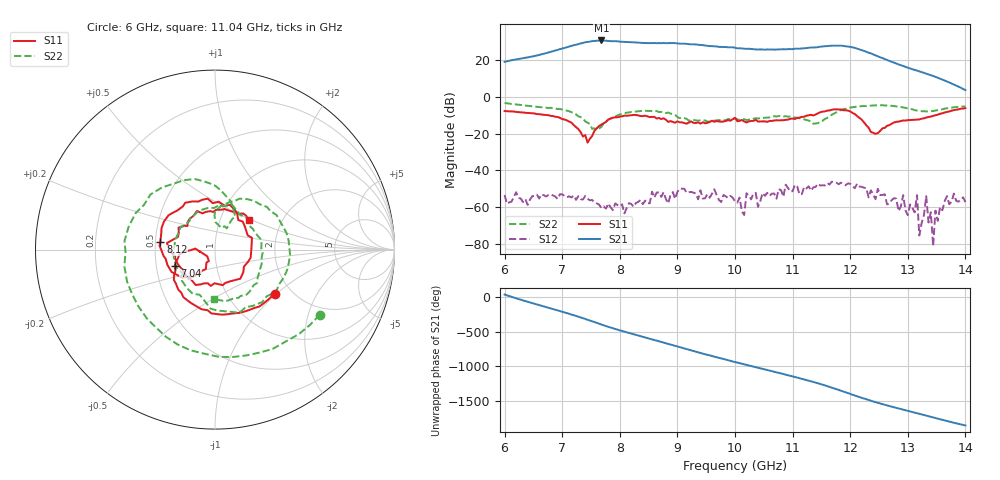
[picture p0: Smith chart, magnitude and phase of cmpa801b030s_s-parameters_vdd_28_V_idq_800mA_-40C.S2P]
!Keysight Technologies,E5071C,MY46110325,B.14.03
!Date: Tue Aug 11 10:33:59 2020
!Data & Calibration Information:
!Freq	S11:SOLT2(ON)	S21:SOLT2(ON)	S12:SOLT2(ON)	S22:SOLT2(ON)
!PortZ  Port1:50+j0  Port2:50+j0
!Above PortZ is port z conversion or system Z0 setting when saving the data.
!When reading, reference impedance value at option line is always used.
# Hz S dB R 50
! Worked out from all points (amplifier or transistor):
!   201 points, 6 GHz to 14 GHz, reference 50 ohm
!   highest |S21| = 30.9 dB at 7.68 GHz (marker M1)
!   |S21| within 3 dB of that: 7.159 GHz to 9.532 GHz (2.373 GHz wide, 28.4 % of centre)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
!   unconditionally stable (mu >= 1): start of sweep to end of sweep
!   at 7.32 GHz: K = 9.67, MAG = 29.7 dB, |S12| = -55.8 dB
!   at 10 GHz: K = 13.75, MAG = 27.5 dB, |S12| = -57.0 dB
!   at 14 GHz: K = 124.67, MAG = 6.6 dB, |S12| = -57.4 dB
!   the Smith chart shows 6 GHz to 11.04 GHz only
!   S11 on the Smith chart (normalised r, x): 6 GHz: 1.64, -0.98; 7.04 GHz: 0.62, -0.12; 8.12 GHz: 0.53, +0.05; 11.04 GHz: 1.36, +0.49
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6e9  -7.63 -36.4  19.18 35.1  -53.50 170.1  -3.26 -31.9
6.56e9  -9.35 -96.8  22.64 -107.2  -53.30 62.6  -5.36 -134.6
7.04e9  -12.26 -157.5  26.77 137.3  -53.99 -12.2  -7.26 122.2
7.36e9  -21.57 -170.9  29.47 52.9  -55.94 -75.2  -11.78 67.5
7.68e9  -15.08 -127.2  30.85 -37.6  -60.60 -168.5  -16.27 89.2
7.88e9  -11.30 -152.8  30.43 -91.1  -61.70 144.4  -11.10 72.4
8.12e9  -10.25 172.3  29.93 -150.5  -60.61 29.2  -8.53 39.3
8.36e9  -10.39 134.1  29.58 152.8  -56.18 -25.6  -7.67 6.8
8.68e9  -11.45 85.6  29.41 78.9  -52.09 -93.2  -8.22 -42.2
9e9  -13.30 17.7  29.24 3.2  -51.82 -148.0  -10.97 -103.6
9.36e9  -13.85 -77.5  28.51 -79.8  -55.81 125.8  -12.91 175.4
9.68e9  -13.15 -131.6  27.59 -150.2  -53.39 28.4  -12.70 114.7
1e10  -11.36 172.2  26.92 138.9  -56.96 -90.5  -11.48 69.0
1.06e10  -13.07 88.5  25.89 16.2  -54.00 -132.8  -11.15 -26.3
1.104e10  -11.99 41.7  26.34 -76.5  -47.94 123.2  -11.23 -91.7
1.136e10  -10.06 9.5  27.01 -149.1  -49.33 82.0  -14.60 -173.1
1.16e10  -7.47 -15.5  27.77 152.7  -46.88 19.0  -11.46 101.6
1.184e10  -6.81 -50.8  28.02 86.3  -46.78 -45.9  -7.15 29.9
1.212e10  -10.43 -104.8  26.38 4.5  -47.33 -153.4  -5.07 -46.3
1.236e10  -19.11 -179.0  23.79 -59.7  -50.92 150.3  -4.70 -101.0
1.268e10  -15.33 52.9  19.67 -135.9  -58.10 114.1  -4.72 -157.1
1.4e10  -6.07 -164.5  3.77 -56.3  -57.36 -45.1  -5.12 -46.3
